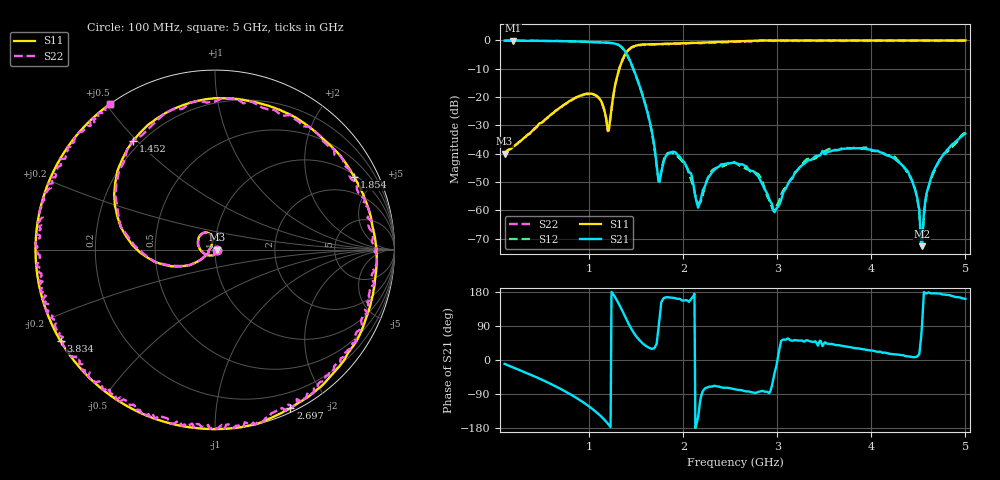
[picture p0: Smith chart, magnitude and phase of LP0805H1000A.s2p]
!	AVX	THIN	FILM	OPERATION
!	LP0805	High	Performance	Low	Pass	Filter	P/N	LP0805H1000ASTR
!	28	June	2017
#	MHz	S	dB	R	50
!	Frq	S11(dB)	S11(deg)	S21(dB)	S21(deg)	S12(dB)	S12(deg)	S22(dB)	S22(deg)
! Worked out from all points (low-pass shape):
!   501 points, 100 MHz to 5 GHz, reference 50 ohm
!   highest |S21| = -0.05 dB at 188.2 MHz (marker M1); lowest = -72.6 dB at 4.539 GHz (marker M2)
!   |S21| within 3 dB of the highest: start of sweep to 1.363 GHz
!   lowest |S11| = -39.9 dB at 100 MHz (marker M3), VSWR 1.02, Z = 51 - j0.0686 ohm
!   |S11| at or under -10 dB: start of sweep to 1.32 GHz
!   |S22| runs from -39.9 to 0.0 dB; largest |S21 - S12| = 0.031
!   S11 on the Smith chart (normalised r, x): 100 MHz: 1.02, -0.00; 1.452 GHz: 0.17, +0.49; 1.854 GHz: 1.09, +3.78; 2.697 GHz: 0.04, -1.58; 3.834 GHz: 0.00, -0.27; 5 GHz: -0.00, +0.51
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100  -39.94 -3.8  -0.07 -10.3  -0.06 -10.0  -39.94 -3.9
188.2  -37.63 -27.8  -0.05 -19.4  -0.06 -19.4  -37.83 -27.8
923.2  -19.25 149.3  -0.42 -109.5  -0.41 -109.6  -19.45 149.3
1207.4  -31.76 159.9  -0.81 -170.7  -0.83 -171.1  -31.76 159.7
1354.4  -6.76 177.1  -2.71 128.5  -2.78 129.4  -6.96 177.1
1452.4  -2.39 126.8  -8.57 80.2  -8.86 78.8  -2.39 126.8
1628.8  -1.36 69.4  -26.71 33.2  -26.55 35.4  -1.56 69.2
1736.6  -1.29 47.1  -49.43 84.7  -49.59 89.6  -1.29 46.9
1854.2  -1.16 27.6  -39.81 165.2  -39.58 164.0  -1.36 27.4
2020.8  -0.98 4.3  -43.63 157.6  -43.95 155.8  -1.08 4.3
2158  -0.82 -12.3  -59.05 -150.3  -57.55 -147.4  -0.82 -12.4
2305  -0.62 -27.9  -46.55 -70.2  -45.89 -72.0  -0.72 -27.9
2550  -0.32 -51.3  -43.33 -77.4  -43.02 -83.7  -0.52 -51.4
2697  -0.19 -64.6  -45.77 -83.1  -45.64 -78.7  -0.39 -64.6
2981.2  0.00 -87.6  -59.94 -24.0  -59.33 -10.1  -0.20 -87.7
3373.2  0.00 -117.0  -41.80 48.0  -41.82 47.5  -0.20 -117.2
3833.8  0.00 -149.3  -38.06 31.1  -37.84 34.1  0.00 -149.4
4186.6  0.00 -173.2  -40.77 16.8  -40.48 16.7  -0.10 -173.4
4431.6  0.00 169.5  -49.45 7.8  -49.34 6.0  -0.20 169.3
4539.4  0.00 161.8  -72.63 93.8  -71.82 103.9  0.00 161.8
4657  0.00 152.9  -46.36 176.2  -47.04 171.5  -0.10 152.7
5000  0.00 125.8  -32.91 161.4  -32.62 158.6  0.00 125.8
